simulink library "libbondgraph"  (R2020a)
settings: Solver=ode45  StartTime=0.0  StopTime=10.0  RelTol=1e-3
undefined symbols (not defined in the file or in its folder): I

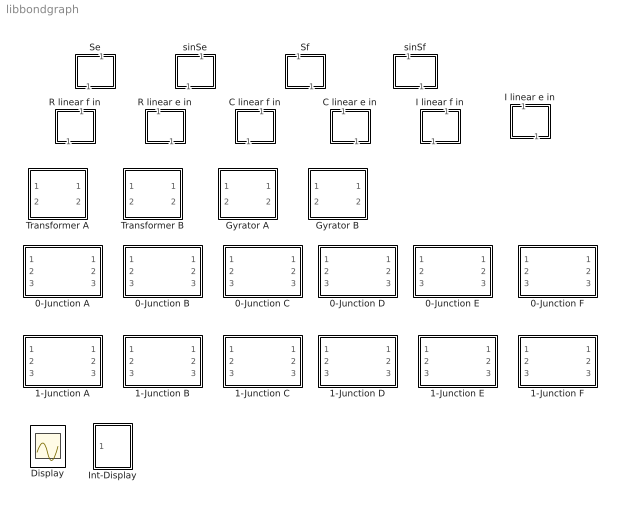
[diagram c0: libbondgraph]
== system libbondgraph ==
  0-Junction A : Subsystem  mask(0-Junction){}
      mask help: 0-Junction Variante A: 3 Bonds rein e2 = e1 e3 = e1 f1 = -f2 - f3
  0-Junction B : Subsystem  mask(0-Junction){}
      mask help: 0-Junction Variante B: 2 Bonds rein, f-kausal bei reingehendem Bond e2 = e1 e3 = e1 f1 = f3 - f2
  0-Junction C : Subsystem  mask(0-Junction){}
      mask help: 0-Junction Variante C: 2 Bonds rein, f-kausal bei rausgehendem Bond e1 = e3 e2 = e3 f3 = f1 + f2
  0-Junction D : Subsystem  mask(0-Junction){}
      mask help: 0-Junction Variante D: 1 Bond rein, f-kausal bei reingehendem Bond e2 = e1 e3 = e1 f1 = f2 + f3
  0-Junction E : Subsystem  mask(0-Junction){}
      mask help: 0-Junction Variante E: 1 Bond rein, f-kausal bei rausgehendem Bond e1 = e3 e2 = e3 f3 = f1 - f2
  0-Junction F : Subsystem  mask(0-Junction){}
      mask help: 0-Junction Variante F: 0 Bonds rein e2 = e1 e3 = e1 f1 = -f2 - f3
  1-Junction A : Subsystem  mask(1-Junction){}
      mask help: 1-Junction Variante A: 3 Bonds rein e1 = -e2 - e3 f2 = f1 f3 = f1
  1-Junction B : Subsystem  mask(1-Junction){}
      mask help: 1-Junction Variante B: 2 Bonds rein, e-kausal bei reingehendem Bond e1 = e3 - e2 f2 = f1 f3 = f1
  1-Junction C : Subsystem  mask(1-Junction){}
      mask help: 1-Junction Variante C: 2 Bonds rein, e-kausal bei rausgehendem Bond e3 = e1 + e2 f1 = f3 f2 = f3
  1-Junction D : Subsystem  mask(1-Junction){}
      mask help: 1-Junction Variante D: 1 Bond rein, e-kausal bei reingehendem Bond e1 = e2 + e3 f2 = f1 f3 = f1
  1-Junction E : Subsystem  mask(1-Junction){}
      mask help: 1-Junction Variante E: 1 Bond rein, e-kausal bei rausgehendem Bond e3 = e1 - e2 f1 = f3 f2 = f3
  1-Junction F : Subsystem  mask(1-Junction){}
      mask help: 1-Junction Variante F: 0 Bonds rein e1 = -e2 - e3 f2 = f1 f3 = f1
  C linear e in : Subsystem  mask(Capacitor, linear){R=1}
      mask help: linear capacitor with incoming effort (differential causality) f = C de/dt
  C linear f in : Subsystem  mask(Capacitor, linear){C=1}
      mask help: linear capacitor with incoming flow (integral causality) e = 1/C int(f dt)
  Display : Scope
  Gyrator A : Subsystem  mask(Gyrator){r=1}
      mask help: Gyrator, Typ A e1 = r f2 e2 = r f1
  Gyrator B : Subsystem  mask(Gyrator){r=1}
      mask help: Gyrator, Typ B f1 = 1/r e2 f2 = 1/r e1
  I linear e in : Subsystem  mask(Inertia, linear){I=1}
      mask help: linear inertia with incoming effort (integral causality) f = 1/I int(e dt)
  I linear f in : Subsystem  mask(Inertia, linear){I=1}
      mask help: linear inertia with incoming flow (differential causality) e = I df/dt
  Int-Display : Subsystem
  R linear e in : Subsystem  mask(Resistor, linear){R=1}
      mask help: linear Resistor with incoming effort f = e / R
  R linear f in : Subsystem  mask(Resistor, linear){R=1}
      mask help: linear Resistor with incoming flow e = R f
  Se : Subsystem  mask(Source of effort){e_ext=1}
      mask prompts: e_ext "Effort"
      mask help: Source of effort, providing a constant effort
  Sf : Subsystem  mask(Source of flow){f_ext=1}
      mask prompts: f_ext "Flow"
      mask help: Source of flow, providing a constant flow
  Transformer A : Subsystem  mask(Tranformer){m=1}
      mask help: Transformer e1 = m e2 f2 = m f1
  Transformer B : Subsystem  mask(Tranformer){m=1}
      mask help: Transformer, Typ B e2 = 1/m e1 f1 = 1/m f2
  sinSe : Subsystem  mask(Source of effort){amplitude=1, frequency=5}
      mask prompts: frequency "Frequenz"
      mask help: Source of effort, providing a effort that changes harmonically with time
  sinSf : Subsystem  mask(Source of flow){amplitude=1, frequency=5}
      mask prompts: frequency "Frequenz"
      mask help: Source of flow, providing a flow that changes harmonically with time

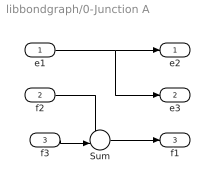
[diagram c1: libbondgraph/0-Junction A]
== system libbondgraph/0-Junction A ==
  e1 : Inport
  f2 : Inport  Port=2
  f3 : Inport  Port=3
  Sum : Sum  Inputs=--|  SaturateOnIntegerOverflow=on
  e2 : Outport
  e3 : Outport  Port=2
  f1 : Outport  Port=3
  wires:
  e1/1 -> e3/1, e2/1
  f3/1 -> Sum/2
  Sum/1 -> f1/1
  f2/1 -> Sum/1

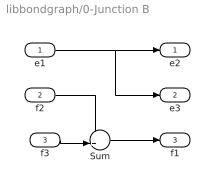
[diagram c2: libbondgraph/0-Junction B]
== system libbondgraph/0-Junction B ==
  e1 : Inport
  f2 : Inport  Port=2
  f3 : Inport  Port=3
  Sum : Sum  Inputs=-+|  SaturateOnIntegerOverflow=on
  e2 : Outport
  e3 : Outport  Port=2
  f1 : Outport  Port=3
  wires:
  f2/1 -> Sum/1
  Sum/1 -> f1/1
  f3/1 -> Sum/2
  e1/1 -> e2/1, e3/1

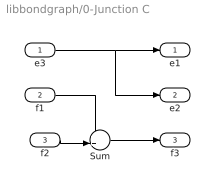
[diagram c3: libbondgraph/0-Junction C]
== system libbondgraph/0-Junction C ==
  e3 : Inport
  f1 : Inport  Port=2
  f2 : Inport  Port=3
  Sum : Sum  Inputs=++|  SaturateOnIntegerOverflow=on
  e1 : Outport
  e2 : Outport  Port=2
  f3 : Outport  Port=3
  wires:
  e3/1 -> e2/1, e1/1
  f2/1 -> Sum/2
  Sum/1 -> f3/1
  f1/1 -> Sum/1

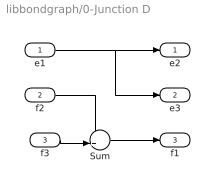
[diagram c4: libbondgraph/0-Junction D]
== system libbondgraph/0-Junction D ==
  e1 : Inport
  f2 : Inport  Port=2
  f3 : Inport  Port=3
  Sum : Sum  Inputs=++|  SaturateOnIntegerOverflow=on
  e2 : Outport
  e3 : Outport  Port=2
  f1 : Outport  Port=3
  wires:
  e1/1 -> e3/1, e2/1
  f3/1 -> Sum/2
  Sum/1 -> f1/1
  f2/1 -> Sum/1

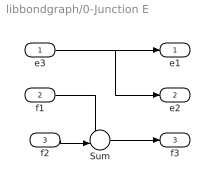
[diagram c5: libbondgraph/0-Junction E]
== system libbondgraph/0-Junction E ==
  e3 : Inport
  f1 : Inport  Port=2
  f2 : Inport  Port=3
  Sum : Sum  Inputs=+-|  SaturateOnIntegerOverflow=on
  e1 : Outport
  e2 : Outport  Port=2
  f3 : Outport  Port=3
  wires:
  f1/1 -> Sum/1
  Sum/1 -> f3/1
  f2/1 -> Sum/2
  e3/1 -> e1/1, e2/1

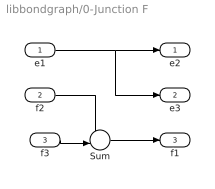
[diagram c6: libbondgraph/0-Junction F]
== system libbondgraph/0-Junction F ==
  e1 : Inport
  f2 : Inport  Port=2
  f3 : Inport  Port=3
  Sum : Sum  Inputs=--|  SaturateOnIntegerOverflow=on
  e2 : Outport
  e3 : Outport  Port=2
  f1 : Outport  Port=3
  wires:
  f2/1 -> Sum/1
  Sum/1 -> f1/1
  f3/1 -> Sum/2
  e1/1 -> e2/1, e3/1

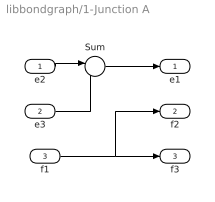
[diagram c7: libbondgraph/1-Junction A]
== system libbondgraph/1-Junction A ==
  e2 : Inport
  e3 : Inport  Port=2
  f1 : Inport  Port=3
  Sum : Sum  Inputs=|--  SaturateOnIntegerOverflow=on
  e1 : Outport
  f2 : Outport  Port=2
  f3 : Outport  Port=3
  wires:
  f1/1 -> f3/1, f2/1
  e2/1 -> Sum/1
  Sum/1 -> e1/1
  e3/1 -> Sum/2

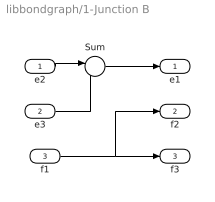
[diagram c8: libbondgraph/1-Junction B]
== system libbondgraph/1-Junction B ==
  e2 : Inport
  e3 : Inport  Port=2
  f1 : Inport  Port=3
  Sum : Sum  Inputs=|-+  SaturateOnIntegerOverflow=on
  e1 : Outport
  f2 : Outport  Port=2
  f3 : Outport  Port=3
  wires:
  e3/1 -> Sum/2
  Sum/1 -> e1/1
  e2/1 -> Sum/1
  f1/1 -> f2/1, f3/1

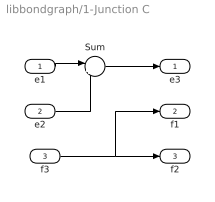
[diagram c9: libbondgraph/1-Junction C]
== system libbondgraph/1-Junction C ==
  e1 : Inport
  e2 : Inport  Port=2
  f3 : Inport  Port=3
  Sum : Sum  Inputs=|++  SaturateOnIntegerOverflow=on
  e3 : Outport
  f1 : Outport  Port=2
  f2 : Outport  Port=3
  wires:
  f3/1 -> f2/1, f1/1
  e1/1 -> Sum/1
  Sum/1 -> e3/1
  e2/1 -> Sum/2

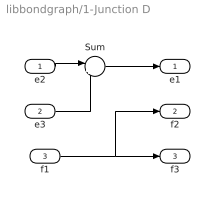
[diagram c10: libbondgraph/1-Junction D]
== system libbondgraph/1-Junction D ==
  e2 : Inport
  e3 : Inport  Port=2
  f1 : Inport  Port=3
  Sum : Sum  Inputs=|++  SaturateOnIntegerOverflow=on
  e1 : Outport
  f2 : Outport  Port=2
  f3 : Outport  Port=3
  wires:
  e3/1 -> Sum/2
  Sum/1 -> e1/1
  e2/1 -> Sum/1
  f1/1 -> f2/1, f3/1

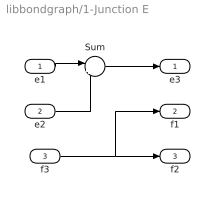
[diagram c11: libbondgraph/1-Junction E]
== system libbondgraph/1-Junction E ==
  e1 : Inport
  e2 : Inport  Port=2
  f3 : Inport  Port=3
  Sum : Sum  Inputs=|+-  SaturateOnIntegerOverflow=on
  e3 : Outport
  f1 : Outport  Port=2
  f2 : Outport  Port=3
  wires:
  f3/1 -> f2/1, f1/1
  e1/1 -> Sum/1
  Sum/1 -> e3/1
  e2/1 -> Sum/2

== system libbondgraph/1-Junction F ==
  e1 : Inport
  e2 : Inport  Port=2
  f3 : Inport  Port=3
  Sum : Sum  Inputs=|+-  SaturateOnIntegerOverflow=on
  e3 : Outport
  f1 : Outport  Port=2
  f2 : Outport  Port=3
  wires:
  e2/1 -> Sum/2
  Sum/1 -> e3/1
  e1/1 -> Sum/1
  f3/1 -> f1/1, f2/1

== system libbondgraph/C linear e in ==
  e : Inport
  Gain : Gain  Gain=1/I  SaturateOnIntegerOverflow=on
  Integrator : Integrator
  f : Outport
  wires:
  e/1 -> Gain/1
  Gain/1 -> Integrator/1
  Integrator/1 -> f/1

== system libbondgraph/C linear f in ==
  f : Inport
  Gain : Gain  Gain=1/C  SaturateOnIntegerOverflow=on
  Integrator : Integrator
  e : Outport
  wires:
  f/1 -> Gain/1
  Gain/1 -> Integrator/1
  Integrator/1 -> e/1

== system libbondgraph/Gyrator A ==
  f1 : Inport
  f2 : Inport  Port=2
  Gain : Gain  Gain=r  SaturateOnIntegerOverflow=on
  Gain1 : Gain  Gain=r  SaturateOnIntegerOverflow=on
  e1 : Outport
  e2 : Outport  Port=2
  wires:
  Gain/1 -> e1/1
  Gain1/1 -> e2/1
  f1/1 -> Gain1/1
  f2/1 -> Gain/1

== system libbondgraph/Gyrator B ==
  e1 : Inport
  e2 : Inport  Port=2
  Gain : Gain  Gain=1/r  SaturateOnIntegerOverflow=on
  Gain1 : Gain  Gain=1/r  SaturateOnIntegerOverflow=on
  f1 : Outport
  f2 : Outport  Port=2
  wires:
  e2/1 -> Gain/1
  e1/1 -> Gain1/1
  Gain1/1 -> f2/1
  Gain/1 -> f1/1

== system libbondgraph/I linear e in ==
  e : Inport
  Gain : Gain  Gain=1/I  SaturateOnIntegerOverflow=on
  Integrator : Integrator
  f : Outport
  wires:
  e/1 -> Gain/1
  Gain/1 -> Integrator/1
  Integrator/1 -> f/1

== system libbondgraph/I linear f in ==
  f : Inport
  Derivative : Derivative
  Gain : Gain  Gain=I  SaturateOnIntegerOverflow=on
  e : Outport
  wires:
  f/1 -> Gain/1
  Gain/1 -> Derivative/1
  Derivative/1 -> e/1

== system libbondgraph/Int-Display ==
  In1 : Inport
  Integrator : Integrator
  Scope : Scope
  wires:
  In1/1 -> Integrator/1
  Integrator/1 -> Scope/1

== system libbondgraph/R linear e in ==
  e : Inport
  Gain : Gain  Gain=1/R  SaturateOnIntegerOverflow=on
  f : Outport
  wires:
  Gain/1 -> f/1
  e/1 -> Gain/1

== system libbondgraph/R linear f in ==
  f : Inport
  Gain : Gain  Gain=R  SaturateOnIntegerOverflow=on
  e : Outport
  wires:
  f/1 -> Gain/1
  Gain/1 -> e/1

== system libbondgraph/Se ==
  f : Inport
  Constant : Constant  Value=e_ext
  Terminator : Terminator
  e : Outport
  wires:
  f/1 -> Terminator/1
  Constant/1 -> e/1

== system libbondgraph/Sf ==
  e : Inport
  Constant : Constant  Value=f_ext
  Terminator : Terminator
  f : Outport
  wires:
  Constant/1 -> f/1
  e/1 -> Terminator/1

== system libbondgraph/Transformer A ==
  e2 : Inport
  f1 : Inport  Port=2
  Gain : Gain  Gain=m  SaturateOnIntegerOverflow=on
  Gain1 : Gain  Gain=m  SaturateOnIntegerOverflow=on
  e1 : Outport
  f2 : Outport  Port=2
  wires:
  Gain1/1 -> f2/1
  Gain/1 -> e1/1
  e2/1 -> Gain/1
  f1/1 -> Gain1/1

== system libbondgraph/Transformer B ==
  e1 : Inport
  f2 : Inport  Port=2
  Gain : Gain  Gain=1/m  SaturateOnIntegerOverflow=on
  Gain1 : Gain  Gain=1/m  SaturateOnIntegerOverflow=on
  e2 : Outport
  f1 : Outport  Port=2
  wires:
  f2/1 -> Gain1/1
  e1/1 -> Gain/1
  Gain/1 -> e2/1
  Gain1/1 -> f1/1

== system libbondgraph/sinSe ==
  f : Inport
  Sine Wave : Sin  Amplitude=amplitude  Frequency=frequency  SampleTime=0
  Terminator : Terminator
  e : Outport
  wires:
  Sine Wave/1 -> e/1
  f/1 -> Terminator/1

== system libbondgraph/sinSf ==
  f : Inport
  Sine Wave : Sin  Amplitude=amplitude  Frequency=frequency  SampleTime=0
  Terminator : Terminator
  e : Outport
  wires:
  f/1 -> Terminator/1
  Sine Wave/1 -> e/1
